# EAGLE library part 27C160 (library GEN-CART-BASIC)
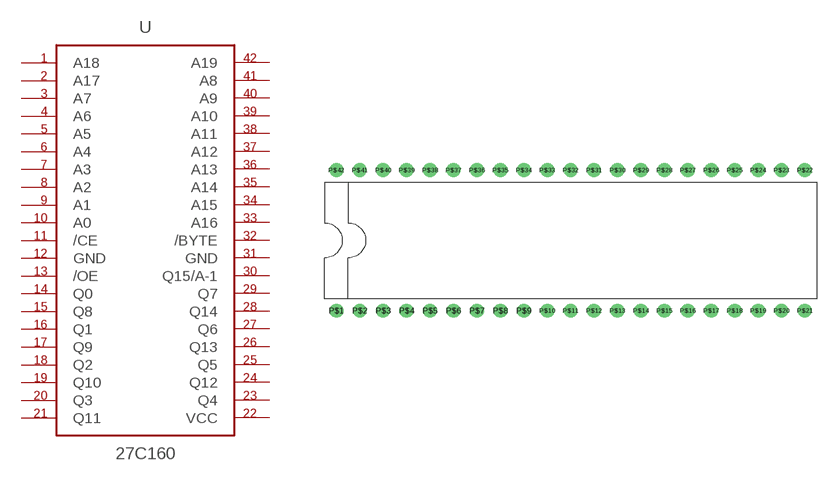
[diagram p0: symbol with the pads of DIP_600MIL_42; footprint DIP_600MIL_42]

Designator prefix U

## 27C160  [DIP_600MIL_42]
P$1  A18  in
P$2  A17  in
P$3  A7  in
P$4  A6  in
P$5  A5  in
P$6  A4  in
P$7  A3  in
P$8  A2  in
P$9  A1  in
P$10  A0  in
P$11  /CE  in
P$12  GND  pwr
P$13  /OE  in
P$14  Q0  out
P$15  Q8  out
P$16  Q1  out
P$17  Q9  out
P$18  Q2  out
P$19  Q10  out
P$20  Q3  out
P$21  Q11  out
P$22  VCC  pwr
P$23  Q4  out
P$24  Q12  out
P$25  Q5  out
P$26  Q13  out
P$27  Q6  out
P$28  Q14  out
P$29  Q7  out
P$30  Q15/A-1
P$31  GND  pwr
P$32  /BYTE  in
P$33  A16  in
P$34  A15  in
P$35  A14  in
P$36  A13  in
P$37  A12  in
P$38  A11  in
P$39  A10  in
P$40  A9  in
P$41  A8  in
P$42  A19  in

## Footprint DIP_600MIL_42 (pad centres in mm)
drill 1: P$1 -25.4,-7.62; P$2 -22.86,-7.62; P$3 -20.32,-7.62; P$4 -17.78,-7.62; P$5 -15.24,-7.62; P$6 -12.7,-7.62; P$7 -10.16,-7.62; P$8 -7.62,-7.62; P$9 -5.08,-7.62; P$10 -2.54,-7.62; P$11 0,-7.62; P$12 2.54,-7.62; P$13 5.08,-7.62; P$14 7.62,-7.62; P$15 10.16,-7.62; P$16 12.7,-7.62; P$17 15.24,-7.62; P$18 17.78,-7.62; P$19 20.32,-7.62; P$20 22.86,-7.62; P$21 25.4,-7.62; P$22 25.4,7.62; P$23 22.86,7.62; P$24 20.32,7.62; P$25 17.78,7.62; P$26 15.24,7.62; P$27 12.7,7.62; P$28 10.16,7.62; P$29 7.62,7.62; P$30 5.08,7.62; P$31 2.54,7.62; P$32 0,7.62; P$33 -2.54,7.62; P$34 -5.08,7.62; P$35 -7.62,7.62; P$36 -10.16,7.62; P$37 -12.7,7.62; P$38 -15.24,7.62; P$39 -17.78,7.62; P$40 -20.32,7.62; P$41 -22.86,7.62; P$42 -25.4,7.62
